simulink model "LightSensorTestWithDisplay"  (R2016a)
settings: Solver=FixedStepAuto  StartTime=0.0  StopTime=inf  RelTol=1e-3
libraries: miniQ x3

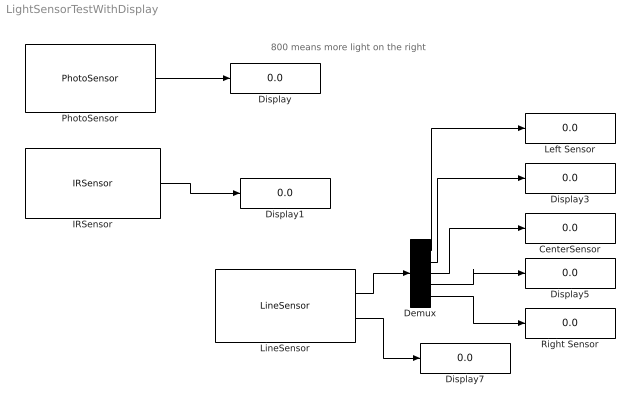
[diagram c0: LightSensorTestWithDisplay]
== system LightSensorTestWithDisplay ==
  note: 800 means more light on the right
  CenterSensor : Display
  Demux : Demux  Outputs=5
  Display{,1,3,5,7} (5 alike) : Display
  IRSensor : miniQ/IRSensor  sampleTime_dd=0.01  debug_dd=off
  Left Sensor : Display
  LineSensor : miniQ/LineSensor  sampleTime_dd=0.01  maxRawSensors=[800,900,900,900,800]  minRawSensors=[200,280,300,300,220]  debug_dd=off
  PhotoSensor : miniQ/PhotoSensor  sampleTime_dd=0.01  debug_dd=off
  Right Sensor : Display
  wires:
  PhotoSensor/1 -> Display/1
  IRSensor/1 -> Display1/1
  LineSensor/1 -> Demux/1
  Demux/5 -> Right Sensor/1
  Demux/4 -> Display5/1
  Demux/3 -> CenterSensor/1
  Demux/2 -> Display3/1
  Demux/1 -> Left Sensor/1
  LineSensor/2 -> Display7/1
